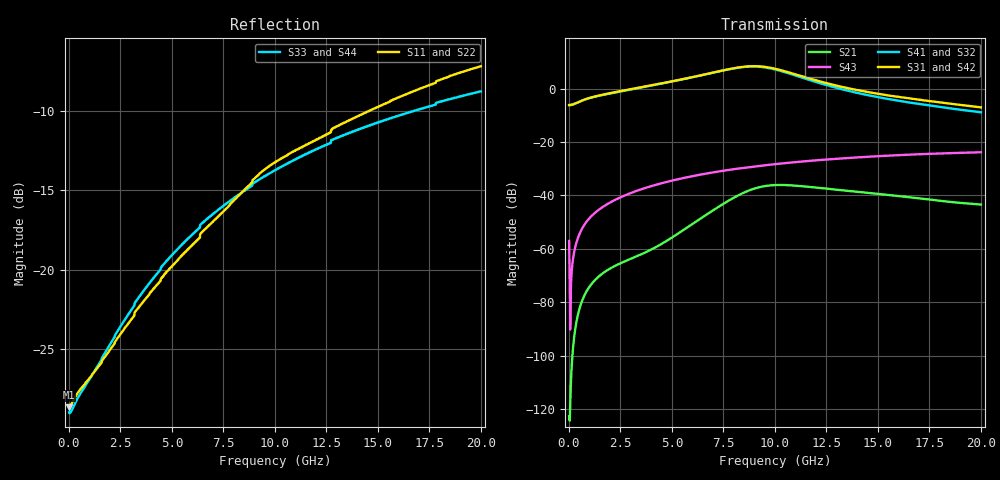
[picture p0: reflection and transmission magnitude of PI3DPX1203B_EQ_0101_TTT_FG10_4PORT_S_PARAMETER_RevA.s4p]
! NPort=4 DATA=2000 NOISE=0 GROUPDELAY=0 COMPLEX_DATAFORMAT=POLAR
! NumOfBlock=1 NumOfParam=0
! .MODEL Smodel S TSTONEFILE=PI3DPX1203B_EQ_0101_TTT_FG10_4PORT_S_PARAMETER_RevA.s4p TYPE=S
!  -- The above .MODEL line can be used for the S element in the netlist.
! The s parameter is extracted from the linear redriver, it is not bi-directional; only s(4,1)s(4,2) and s(3,1)s(3,2)
! should be the insertion loss
!Port definition:
!Port1 = input+
!Port2 = input-
!Port3 = output+
!Port4 = output-
# Hz S MA R  50
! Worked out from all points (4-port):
!   2000 points, 10 MHz to 20 GHz, reference 50 ohm
!   strongest paths, dB at 10 MHz, 5.01 GHz, 10.01 GHz, 15.01 GHz, 20 GHz:
!     S31: -6.2, 2.7, 7.4, -1.9, -7.0
!     S42: -6.2, 2.7, 7.4, -1.9, -7.0
!     S41: -6.2, 2.7, 7.2, -3.2, -8.9
!     S32: -6.2, 2.7, 7.2, -3.2, -8.8
!     S43: -57.1, -34.4, -28.3, -25.3, -23.8
!     S21: -122.7, -55.7, -36.1, -39.4, -43.4
!   lowest |S11| = -28.6 dB at 10 MHz (marker M1), VSWR 1.08, Z = 46.4 - j0.0306 ohm
!   |S11| at or under -10 dB: start of sweep to 14.59 GHz
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1e7  0.03701 -179.5  7.338e-07 10.6  0 0.0  0 0.0
     7.338e-07 10.6  0.03701 -179.5  0 0.0  0 0.0
     0.4917 -0.1  0.4917 179.9  0.03566 178.2  0.001403 -77.8
     0.4917 179.9  0.4917 -0.1  0.001403 -77.8  0.03566 178.2
1.57e9  0.05094 -144.8  0.0003314 115.8  5.133e-12 74.5  4.908e-11 115.4
        0.0003314 115.8  0.05094 -144.8  4.908e-11 115.4  5.133e-12 74.5
        0.7586 6.6  0.7517 -173.4  0.05202 -142.1  0.005823 82.8
        0.7517 -173.4  0.7586 6.6  0.005823 82.8  0.05202 -142.1
6.11e9  0.1218 -110.9  0.003129 143.1  1.664e-08 -116.8  1.482e-07 66.5
        0.003128 143.2  0.1218 -110.9  1.481e-07 66.5  1.664e-08 -116.8
        1.675 -45.2  1.673 136.8  0.1312 -116.9  0.02343 64.6
        1.673 136.8  1.675 -45.2  0.02343 64.6  0.1312 -116.9
8.51e9  0.1779 -105.6  0.01137 107.6  3.931e-07 157.3  1.085e-06 17.0
        0.01136 107.7  0.1779 -105.6  1.084e-06 17.0  3.933e-07 157.3
        2.574 -100.8  2.545 80.9  0.1769 -115.9  0.03301 52.3
        2.546 80.9  2.573 -100.8  0.03301 52.3  0.1769 -115.9
9.98e9  0.217 -107.3  0.01564 64.7  1.249e-06 95.5  2.138e-06 -20.6
        0.01562 64.8  0.217 -107.2  2.135e-06 -20.5  1.25e-06 95.6
        2.37 -148.9  2.3 32.5  0.2051 -116.3  0.03842 44.5
        2.302 32.5  2.368 -148.9  0.03842 44.5  0.2051 -116.3
1.212e10  0.2585 -108.9  0.01391 22.8  3.057e-06 30.5  3.895e-06 -48.4
          0.01389 22.9  0.2585 -108.8  3.895e-06 -48.2  3.059e-06 30.5
          1.385 165.5  1.286 -12.6  0.2414 -117.5  0.04583 33.5
          1.288 -12.6  1.384 165.5  0.04583 33.5  0.2414 -117.5
2e10  0.4365 -116.9  0.006719 -19.4  2.212e-05 -107.3  3.208e-05 -133.9
      0.006753 -19.0  0.4366 -116.9  3.216e-05 -133.9  2.215e-05 -107.2
      0.4461 80.9  0.3613 -83.2  0.3637 -123.9  0.06431 -7.1
      0.361 -83.3  0.4468 80.9  0.06431 -7.1  0.3637 -123.9
